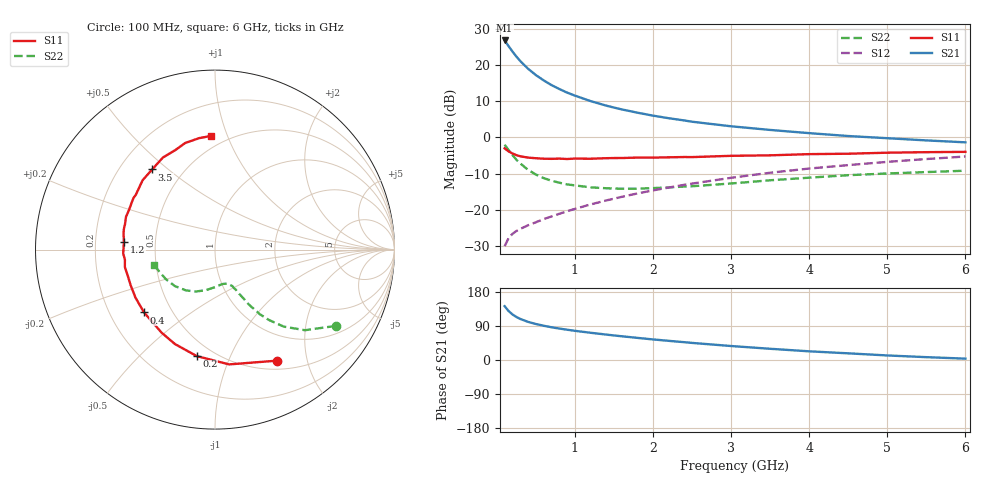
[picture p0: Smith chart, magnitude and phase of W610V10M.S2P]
! SIEMENS Small Signal Semiconductors
! BFR193W
! Si NPN RF Bipolar Junction Transistor in SOT323
! VCE = 10 V  IC = 10 mA
! Common Emitter S-Parameters:  September  1992
# GHz  S  MA  R  50
!  f  S11  S21  S12  S22
! GHz  MAG  ANG  MAG  ANG  MAG  ANG  MAG  ANG
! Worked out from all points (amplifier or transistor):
!   28 points, 100 MHz to 6 GHz, reference 50 ohm
!   highest |S21| = 26.7 dB at 100 MHz (marker M1)
!   |S21| within 3 dB of that: start of sweep to 199.1 MHz
!   unconditionally stable (mu >= 1): 1.054 GHz to 2.635 GHz
!   at 300 MHz: K = 0.54, MSG = 23.1 dB, |S12| = -25.2 dB
!   at 1.5 GHz: K = 1.05, MAG = 11.2 dB, |S12| = -16.9 dB
!   at 6 GHz: K = 0.88, MSG = 2.0 dB, |S12| = -5.2 dB
!   S11 on the Smith chart (normalised r, x): 100 MHz: 0.61, -1.52; 200 MHz: 0.41, -0.76; 400 MHz: 0.35, -0.34; 1.2 GHz: 0.33, +0.04; 3.5 GHz: 0.34, +0.44; 6 GHz: 0.41, +0.87
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0.1  0.7083 -60.9  21.7 142.1  0.0318 62.6  0.7959 -32.3
0.15  0.6444 -83.0  18.17 129.5  0.0409 55.5  0.6725 -41.9
0.2  0.602 -99.7  15.32 120.3  0.0469 51.8  0.5741 -48.3
0.25  0.5717 -112.9  13.05 113.7  0.0514 49.9  0.4947 -52.5
0.3  0.5503 -122.7  11.32 108.4  0.055 49.2  0.4392 -55.2
0.4  0.528 -138.5  8.845 100.6  0.0617 49.7  0.3583 -58.4
0.5  0.5176 -148.9  7.238 95.0  0.0679 51.4  0.3085 -60.0
0.6  0.5101 -157.2  6.116 90.4  0.075 53.3  0.2753 -61.6
0.7  0.5074 -163.5  5.267 86.4  0.0816 54.9  0.2536 -62.5
0.8  0.5115 -169.0  4.655 83.0  0.0888 56.6  0.2382 -63.8
0.9  0.505 -173.7  4.152 79.9  0.0964 58.0  0.2259 -64.5
1  0.5119 -177.5  3.774 77.0  0.1037 59.1  0.2186 -65.9
1.2  0.5093 175.2  3.174 71.9  0.1194 60.7  0.2054 -68.9
1.4  0.5181 169.6  2.748 67.1  0.1355 61.8  0.1997 -72.1
1.6  0.5209 164.3  2.437 62.6  0.152 62.4  0.1964 -75.6
1.8  0.5284 159.8  2.195 58.4  0.1694 62.7  0.1972 -79.6
2.2  0.5327 150.8  1.842 50.6  0.2042 62.2  0.2048 -87.0
3  0.5587 136.2  1.426 36.9  0.2781 59.3  0.2322 -102.9
3.5  0.5675 128.1  1.27 29.6  0.3268 56.1  0.2572 -114.7
4.5  0.5972 111.6  1.047 17.6  0.4161 48.3  0.3022 -137.7
5.5  0.6273 98.0  0.911 7.5  0.5044 40.1  0.3337 -158.2
6  0.6336 92.1  0.857 3.6  0.5468 35.3  0.3483 -165.5
